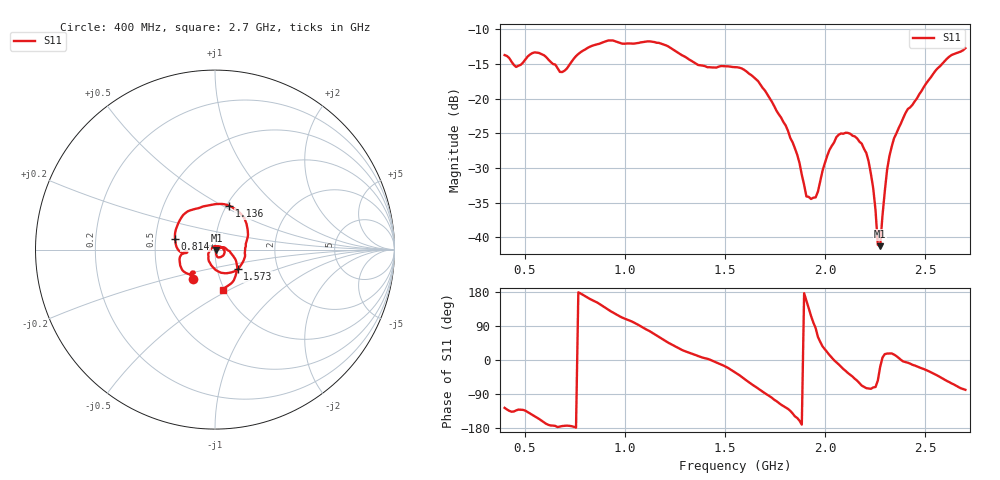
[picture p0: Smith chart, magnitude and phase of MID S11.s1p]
!Keysight Technologies,E5080B,MY59100498,A.17.05.10
!Date: Tuesday, August 29, 2023 17:57:46
!Correction: S11(C  1-Port  )
!S1P File: Measurement: S11:
# Hz S  dB  R 50
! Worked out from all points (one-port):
!   201 points, 400 MHz to 2.7 GHz, reference 50 ohm
!   lowest |S11| = -41.3 dB at 2.275 GHz (marker M1), VSWR 1.02, Z = 50.8 - j0.278 ohm
!   |S11| at or under -10 dB: start of sweep to end of sweep
!   S11 on the Smith chart (normalised r, x): 400 MHz: 0.75, -0.26; 814 MHz: 0.63, +0.08; 1.136 GHz: 1.03, +0.54; 1.573 GHz: 1.26, -0.28; 2.7 GHz: 0.98, -0.47
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4e8  -13.74 -126.2
4.575e8  -15.45 -133.0
5.725e8  -13.44 -155.7
6.875e8  -16.18 -174.3
8.14e8  -12.71 164.5
9.75e8  -11.99 115.1
1.136e9  -11.81 72.1
1.2625e9  -13.36 32.4
1.55e9  -15.48 -32.8
1.573e9  -15.56 -40.4
1.6995e9  -18.85 -87.8
1.8375e9  -26.30 -141.0
1.9065e9  -34.10 156.8
1.9295e9  -34.46 116.3
1.9525e9  -34.23 84.3
2.01e9  -28.27 20.2
2.056e9  -25.56 -5.9
2.125e9  -25.06 -39.1
2.1825e9  -26.50 -67.4
2.217e9  -29.07 -75.2
2.24e9  -32.93 -72.4
2.263e9  -41.06 -54.1
2.2745e9  -41.25 -18.4
2.2975e9  -33.42 15.5
2.3205e9  -28.33 17.3
2.4125e9  -21.51 -7.1
2.562e9  -15.63 -41.5
2.7e9  -12.75 -78.7
